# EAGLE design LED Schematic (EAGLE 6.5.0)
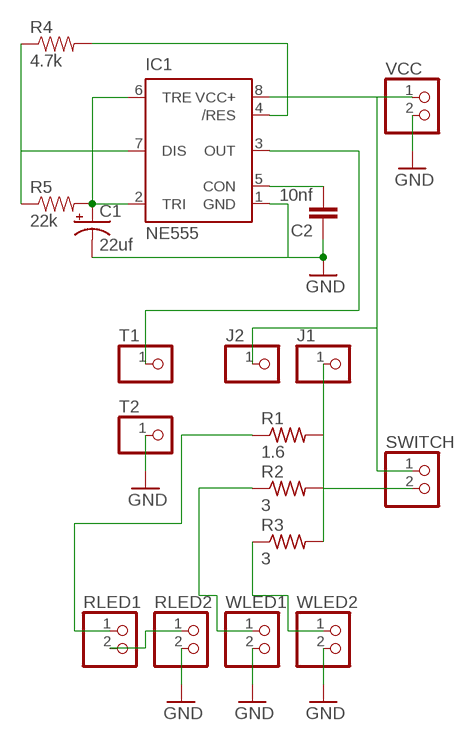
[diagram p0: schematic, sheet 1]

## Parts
C1  22uf  CPOL-USE1,8-4C  [E1,8-4]
C2  10nf  C2.5/2  [C2.5-2]
IC1  NE555  [DIL-08]
J1  PINHD-1X1  [1X01]
J2  PINHD-1X1  [1X01]
R1  1.6  R-US_0617/17C  [0617/17]
R2  3  R-US_0617/17C  [0617/17]
R3  3  R-US_0617/17C  [0617/17]
R4  4.7k  RESISTORKIT  [AXIAL-0.3-KIT]
R5  22k  RESISTORKIT  [AXIAL-0.3-KIT]
RLED1  PINHD-1X2  [1X02]
RLED2  PINHD-1X2  [1X02]
SWITCH  PINHD-1X2  [1X02]
T1  PINHD-1X1  [1X01]
T2  PINHD-1X1  [1X01]
VCC  PINHD-1X2  [1X02]
WLED1  PINHD-1X2  [1X02]
WLED2  PINHD-1X2  [1X02]

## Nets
GND: C1.- C2.1 IC1.1(GND) RLED2.2 T2.1 VCC.2 WLED1.2 WLED2.2
N$1: J1.1 R1.2 R2.2 R3.2 SWITCH.2
N$2: IC1.7(DIS) R4.P$1 R5.P$1
N$3: C1.+ IC1.2(TRI) IC1.6(TRE) R5.P$2
N$4: IC1.4(/RES) IC1.8(VCC+) J2.1 R4.P$2 SWITCH.1 VCC.1
N$5: R1.1 RLED1.1
N$6: C2.2 IC1.5(CON)
N$7: IC1.3(OUT) T1.1
N$8: RLED1.2 RLED2.1
N$9: R2.1 WLED1.1
N$10: R3.1 WLED2.1

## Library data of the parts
C1 = rcl:CPOL-US: POLARIZED CAPACITOR, American symbol
C2 = capacitor-wima:C: CAPACITOR
IC1 = st-microelectronics:NE555: General purpose bipolar Timer; MF: Arrow Electronics; MPN: NE555N; OC_FARNELL: 1467742; OC_NEWARK: 89K1486
J1 J2 T1 T2 = pinhead:PINHD-1X1: PIN HEADER
R1-R3 = resistor:R-US_: RESISTOR, American symbol
R4 R5 = SparkFun-Passives:RESISTOR: Resistor
RLED1 RLED2 SWITCH VCC WLED1 WLED2 = pinhead:PINHD-1X2: PIN HEADER

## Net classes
0 default: width 0.381 mm, drill 0.508 mm, clearance 0.381 mm

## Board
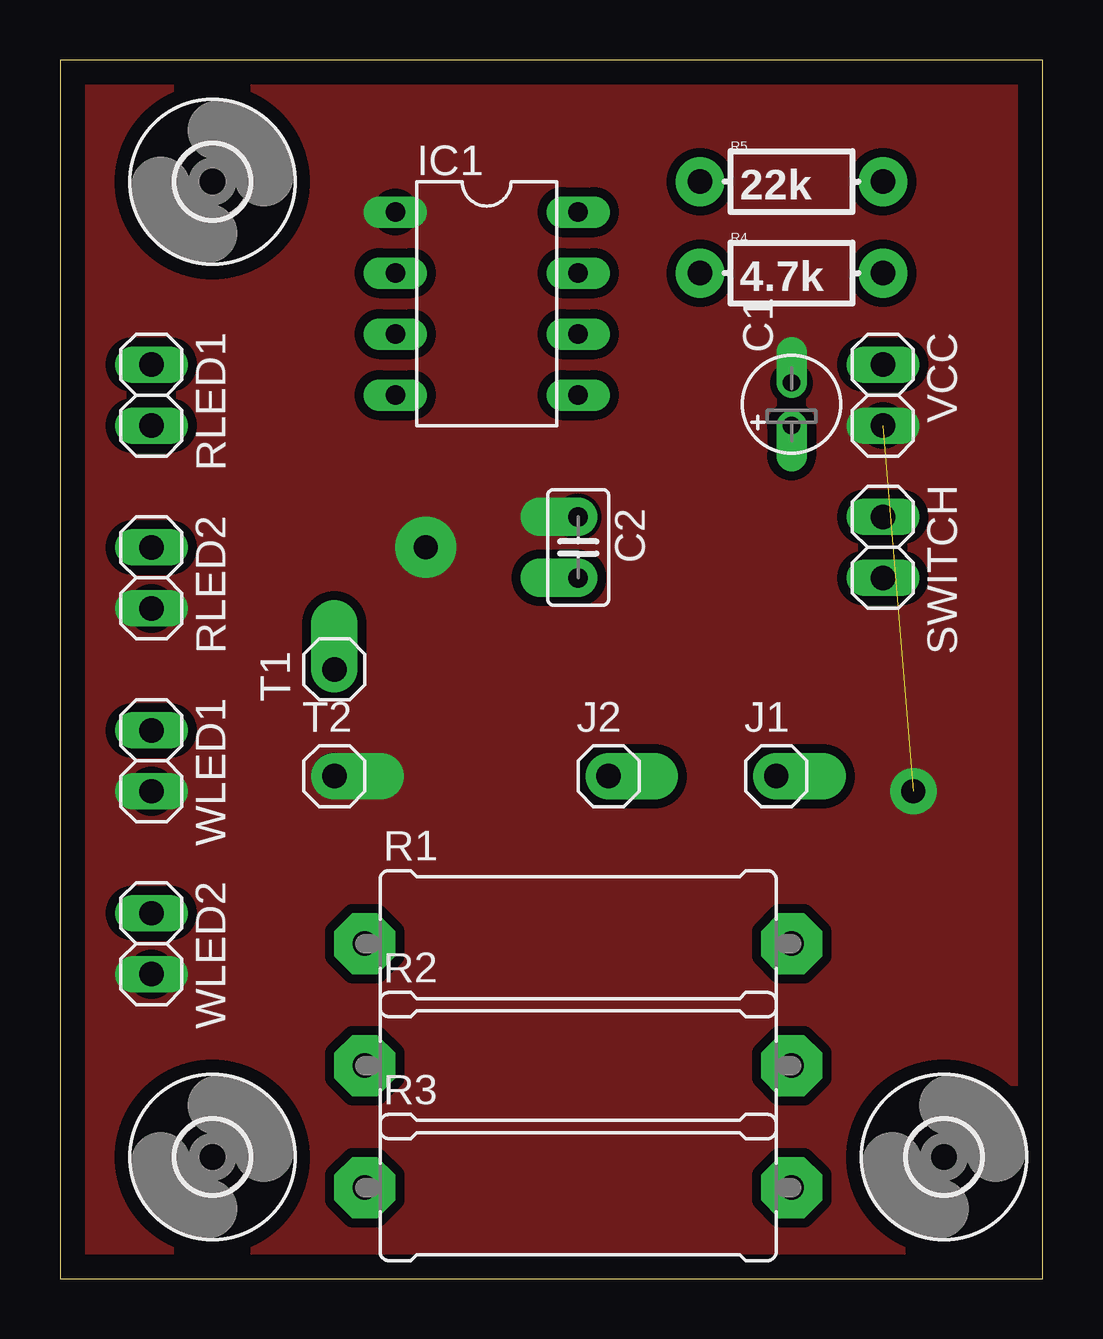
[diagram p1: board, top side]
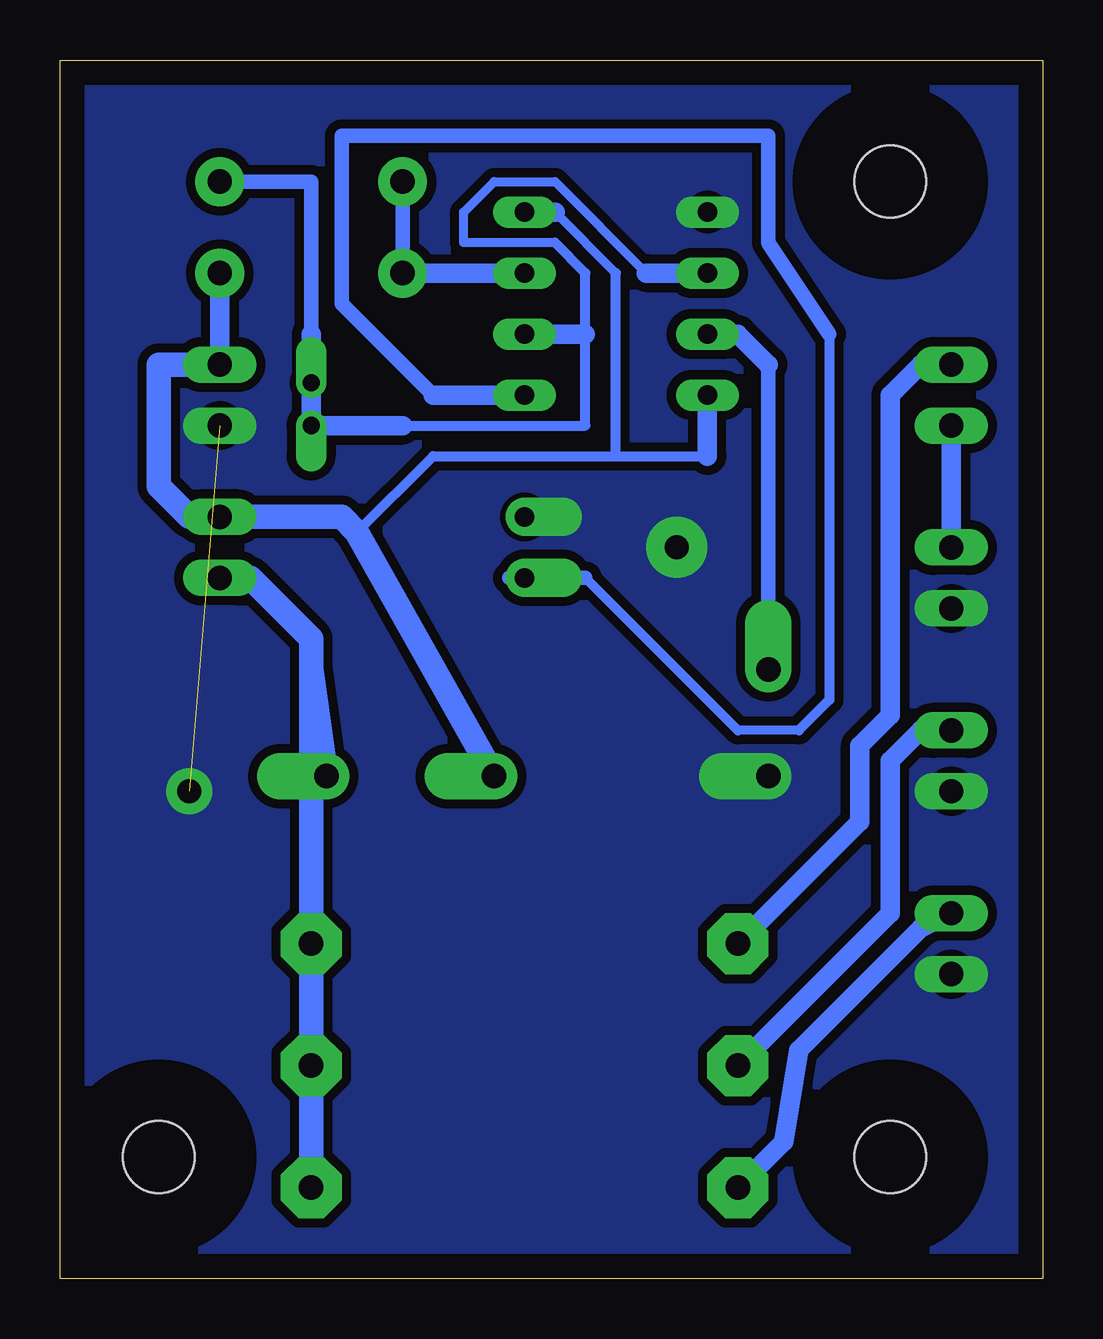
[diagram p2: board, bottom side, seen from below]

Size 40.95 x 50.79 mm. Coordinates in mm from the lower left corner, seen from the top.
Outline: 0,0 40.95,0 40.95,50.79 0,50.79 0,0
Copper layers (1*16): Top 0.035mm / dielectric 1.5mm / Bottom 0.035mm
Design rules "default": minimum track width 10mil, minimum drill 24mil, track to track 8mil, track to pad 8mil, pad to pad 8mil, via to via 8mil, smd to smd 8mil, copper to edge 40mil, drill to drill 8mil, minimum pad ring 10mil, minimum via ring 8mil, stop-mask expansion 4mil, vias tented up to drill 0mil, thermal gap 10mil

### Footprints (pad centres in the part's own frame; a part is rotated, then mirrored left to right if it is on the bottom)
E1,8-4 = drill 0.711 pad 1.27 offset: + -0.889,0; - 0.889,0
C2.5-2 = drill 0.813 pad 1.6 offset: 1 -1.27,0; 2 1.27,0
DIL-08 = drill 0.813 long: 1 -3.81,-3.81; 2 -1.27,-3.81; 3 1.27,-3.81; 4 3.81,-3.81; 5 3.81,3.81; 6 1.27,3.81; 7 -1.27,3.81; 8 -3.81,3.81
1X01 = drill 1.016 pad 1.93 offset: 1 0,0
0617/17 = drill 1.016 pad 2.54 octagon: 1 -8.89,0; 2 8.89,0
AXIAL-0.3-KIT = drill 1.016 pad 2.032: P$1 -3.81,0; P$2 3.81,0
1X02 = drill 1.016 long: 1 -1.27,0; 2 1.27,0
3,0 = hole 3: 0,0

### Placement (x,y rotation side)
C1  30.48,36.45 90 top
C2  21.59,30.48 270 top
IC1  17.78,40.64 270 top
J1  29.84,20.95 0 top
J2  22.86,20.95 0 top
R1  21.59,13.97 0 top
R2  21.59,8.89 0 top
R3  21.59,3.81 0 top
R4  30.48,41.91 0 top
R5  30.48,45.72 0 top
RLED1  3.81,36.83 270 top
RLED2  3.81,29.21 270 top
SWITCH  34.29,30.48 270 top
T1  11.43,25.4 90 top
T2  11.43,20.95 0 top
U$1  [3,0]  6.35,5.08 0 top
U$2  [3,0]  6.35,45.72 0 top
U$3  [3,0]  36.83,5.08 0 top
VCC  34.29,36.83 270 top
WLED1  3.81,21.59 270 top
WLED2  3.81,13.97 270 top

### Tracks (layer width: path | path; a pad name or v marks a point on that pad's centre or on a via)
GND  (via drill 1 pad 1.93, 1 pad 2.54)  (1 unrouted)
  other vias: 15.24,30.48 35.56,20.32
  pour Bottom (no thermals): -2.54,53.34 43.18,53.34 43.18,-2.54 -2.54,-2.54
  pour Top (no thermals): -2.54,53.34 43.18,53.34 43.18,-2.54 -2.54,-2.54
N$1
  Bottom 1.016: 30.48,25.4 30.48,26.67 33.02,29.21 SWITCH.2 | R3.2 R2.2 R1.2 30.48,25.4 | 30.48,25.4 J1.1
N$2
  Bottom 0.61: R4.P$1 R5.P$1
  Bottom 0.813: R4.P$1 IC1.7
N$3
  Bottom 0.381: 16.51,41.91 20.32,45.72 22.86,45.72 24.13,44.45 24.13,43.18 20.32,43.18
  Bottom 0.406: 26.67,35.56 19.05,35.56 19.05,39.37 19.05,41.91 20.32,43.18
  Bottom 0.61: R5.P$2 30.48,45.72 30.48,39.37
  Bottom 0.813: 26.67,35.56 C1.+ 30.48,39.37 | 16.51,41.91 IC1.2 | 19.05,39.37 IC1.6
N$4
  Bottom 0.381: 17.78,41.91 20.32,44.45
  Bottom 0.406: 17.78,34.29 25.4,34.29 28.57,31.11 | 17.78,34.29 13.97,34.29 | 17.78,34.29 17.78,41.91
  Bottom 0.813: R4.P$2 VCC.1 | 13.97,34.29 IC1.4 | 20.32,44.45 IC1.8
  Bottom 1.016: VCC.1 36.83,38.1 36.83,33.02 35.56,31.75 SWITCH.1 29.21,31.75 28.57,31.11 J2.1
N$5
  Bottom 0.813: RLED1.1 5.08,38.1 6.35,36.83 6.35,23.5 7.62,22.23 7.62,19.05 R1.1
N$6
  Bottom 0.381: 10.16,22.86 12.7,22.86
  Bottom 0.406: 12.7,22.86 19.05,29.21 | 8.89,39.37 8.89,24.13 10.16,22.86
  Bottom 0.61: 19.05,29.21 C2.2 22.23,29.21 | 8.89,39.37 11.43,43.18 11.43,47.62 29.21,47.62 29.21,40.64 25.4,36.83
  Bottom 0.813: IC1.5 25.4,36.83
N$7
  Bottom 0.61: T1.1 11.43,38.1
  Bottom 0.813: IC1.3 12.7,39.37 11.43,38.1
N$8
  Bottom 0.813: RLED1.2 RLED2.1
N$9
  Bottom 0.813: WLED1.1 5.08,22.86 6.35,21.59 6.35,15.24 R2.1
N$10
  Bottom 0.813: R3.1 10.79,5.71 10.16,9.53 5.08,14.61 WLED2.1
(copper drawn outside any net)
  shapes: Bottom circle x10, Top circle x10

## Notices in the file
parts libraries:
SparkFun-Passives: Licensing: CC v3.0 Share-Alike You are welcome to use this library for commercial purposes.
